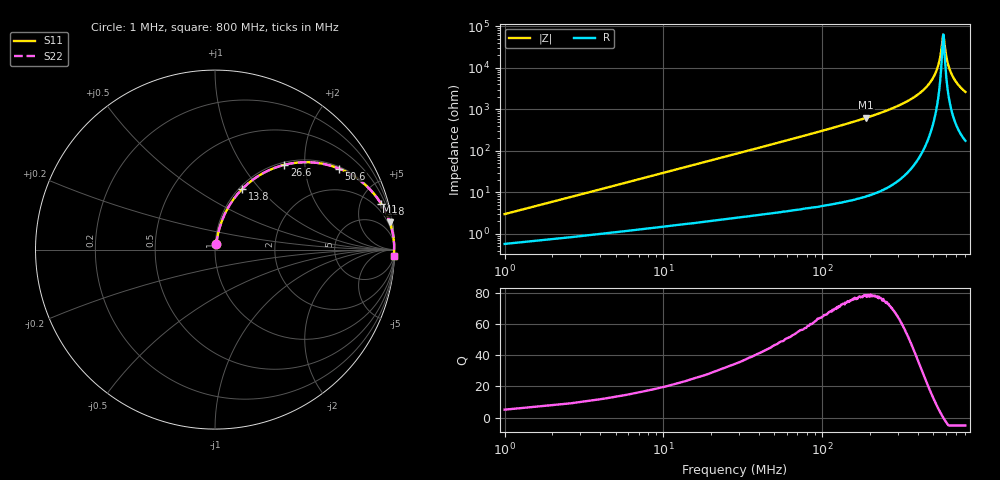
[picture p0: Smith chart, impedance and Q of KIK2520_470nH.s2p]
!version-2
!date-01.2022
!Series
# MHz S RI R 50
!Freq ReS11 ImS11 ReS21 ImS21 ReS12 ImS12 ReS22 ImS22
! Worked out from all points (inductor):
!   501 points, 1 MHz to 800 MHz, reference 50 ohm
!   read as one part in series: L = 470 nH near 4.2 MHz
!   highest Q = 78.4 at 190 MHz (marker M1), where L = 526 nH
!   self-resonance near 580 MHz
!   S11 on the Smith chart (normalised r, x): 1 MHz: 1.01, +0.06; 13.8 MHz: 1.03, +0.82; 26.6 MHz: 1.05, +1.57; 50.6 MHz: 1.06, +3.01; 118 MHz: 1.11, +7.26; 800 MHz: 5, -52
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1  0.00657 0.0292  0.9934 -0.0292  0.9934 -0.0292  0.00657 0.0292
7.4  0.0568 0.2035  0.9432 -0.2035  0.9432 -0.2035  0.0568 0.2035
13.8  0.1531 0.3394  0.8469 -0.3394  0.8469 -0.3394  0.1531 0.3394
26.6  0.3861 0.4721  0.6139 -0.4721  0.6139 -0.4721  0.3861 0.4721
50.6  0.6903 0.4518  0.3097 -0.4518  0.3097 -0.4518  0.6903 0.4518
77.8  0.8413 0.3568  0.1587 -0.3568  0.1587 -0.3568  0.8413 0.3568
118  0.9262 0.2542  0.0737 -0.2542  0.0737 -0.2542  0.9262 0.2542
135  0.9443 0.2226  0.0557 -0.2226  0.0557 -0.2226  0.9443 0.2226
190  0.9734 0.1548  0.0266 -0.1548  0.0266 -0.1548  0.9734 0.1548
268  0.9889 0.0981  0.0111 -0.0981  0.0111 -0.0981  0.9889 0.0981
401  0.9969 0.044  0.00313 -0.044  0.00313 -0.044  0.9969 0.044
483  0.9982 0.0216  0.00178 -0.0216  0.00178 -0.0216  0.9982 0.0216
534  0.9985 0.0098  0.00153 -0.0098  0.00153 -0.0098  0.9985 0.0098
555  0.9985 0.00535  0.00152 -0.00535  0.00152 -0.00535  0.9985 0.00535
580  0.9984 0.000102  0.00157 -0.000102  0.00157 -0.000102  0.9984 0.000102
587  0.9984 -0.00117  0.00159 0.00117  0.00159 0.00117  0.9984 -0.00117
599  0.9984 -0.00368  0.00165 0.00368  0.00165 0.00368  0.9984 -0.00368
615  0.9983 -0.00674  0.00174 0.00674  0.00174 0.00674  0.9983 -0.00674
639  0.9981 -0.0112  0.00191 0.0112  0.00191 0.0112  0.9981 -0.0112
667  0.9978 -0.0161  0.00215 0.0161  0.00215 0.0161  0.9978 -0.0161
719  0.9972 -0.025  0.00276 0.025  0.00276 0.025  0.9972 -0.025
800  0.996 -0.0377  0.00396 0.0377  0.00396 0.0377  0.996 -0.0377
